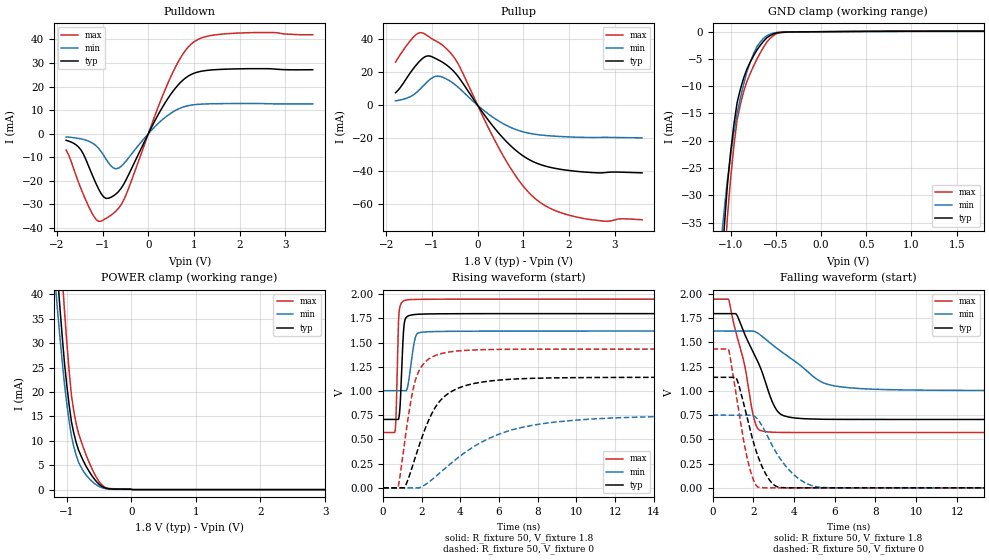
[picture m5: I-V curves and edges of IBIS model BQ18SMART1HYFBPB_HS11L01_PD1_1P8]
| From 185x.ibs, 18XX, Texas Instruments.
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|   Model Cell BQ18SMART1HYFBPB_HS11L01_PD1_1P8
|BQ18SMART1HYFBPB_HS11L01_PD1_1P8
[Model]   BQ18SMART1HYFBPB_HS11L01_PD1_1P8
Model_type   I/O
Polarity   Non-Inverting
Enable   Active-Low
Vinl =  0.63
Vinh =  1.17
Cref =  15pF
Rref =  100.0000M
Vref =  0V
Vmeas =  0.9
C_comp   0.915143p   0.8088923p   1.028577p
[Model Spec]
Vinl   0.63   0.567   0.6825
Vinh   1.17   1.053   1.2675
[Temperature Range]   25   125   -40
[Voltage Range]   1.8   1.62   1.95
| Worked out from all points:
|   slope of the pulldown table from 0 to 0.27 V, typ, clamps not added: 27.2 ohm
|   slope of the pullup table from 0 to 0.27 V, typ, clamps not added: 26 ohm
|   GND clamp passes 1 mA (typ) near -0.59 V on its own axis
|   POWER clamp passes 1 mA (typ) near -0.49 V on its own axis
|   rising waveform, R_fixture 50, V_fixture 1.8: 20-80 % time 144ps typ, 263ps min, 101ps max; typ from 0.706 V to 1.8 V
|   rising waveform, R_fixture 50, V_fixture 0: 20-80 % time 1.49ns typ, 3.72ns min, 739ps max; typ from 0 V to 1.14 V
|   falling waveform, R_fixture 50, V_fixture 1.8: 20-80 % time 1.27ns typ, 2.26ns min, 837ps max; typ from 1.8 V to 0.706 V
|   falling waveform, R_fixture 50, V_fixture 0: 20-80 % time 937ps typ, 1.39ns min, 707ps max; typ from 1.14 V to 0 V
| Nom Voltages:
|   BIASFET=1.8, VBBNW=1.1, VDD=1.1, VDDS=1.8, VSS=0, VSSS=0
| Min Voltages:
|   BIASFET=1.62, VBBNW=0.99, VDD=0.99, VDDS=1.62, VSS=0, VSSS=0
| Max Voltages:
|   BIASFET=1.95, VBBNW=1.21, VDD=1.21, VDDS=1.95, VSS=0, VSSS=0
[POWER_clamp]
|   voltage   I(typ)   I(min)   I(max)
-1.8V     196.9mA    157.5mA    250.4mA
-1.182V   51.67mA    43mA       68.61mA
-1.145V   44.45mA    37.16mA    60.1mA
-1.109V   37.9mA     31.74mA    52.07mA
-1.073V   31.79mA    26.6mA     44.33mA
-1.036V   26.12mA    21.74mA    36.87mA
-963.6mV  17.39mA    14.07mA    24.42mA
-927.3mV  13.91mA    10.96mA    19.29mA
-854.5mV  9.657mA    7.054mA    13.5mA
-709.1mV  4.995mA    3.131mA    7.393mA
-490.9mV  991uA      585.4uA    1.466mA
3.6V      0A         0A         0A
[Pulldown]
|   voltage   I(typ)   I(min)   I(max)
-1.8V     -2.835mA   -1.376mA   -6.938mA
-1.473V   -6.994mA   -2.229mA   -23.44mA
-1.2V     -18.79mA   -4.282mA   -34.89mA
-1.036V   -25.34mA   -7.531mA   -37.14mA
-872.7mV  -27.39mA   -12.36mA   -35.28mA
-654.5mV  -24.59mA   -14.63mA   -31.68mA
-490.9mV  -19.69mA   -11.65mA   -26.08mA
381.8mV   13.54mA    7.116mA    19.32mA
654.5mV   20.72mA    10.44mA    30.47mA
927.3mV   25mA       12.07mA    37.79mA
1.636V    27.3mA     12.74mA    42.26mA
3.6V      27.12mA    12.64mA    41.97mA
[Pullup]
|   voltage   I(typ)   I(min)   I(max)
-1.8V     7.614mA    2.74mA     26.22mA
-1.527V   17.69mA    4.626mA    37.43mA
-1.309V   25.69mA    8.541mA    43.72mA
-1.036V   29.87mA    15.94mA    41.05mA
-818.2mV  26.95mA    17.52mA    37.49mA
-490.9mV  19.61mA    12.45mA    28.08mA
545.5mV   -19.54mA   -10.94mA   -30.03mA
927.3mV   -29.38mA   -15.56mA   -46.58mA
1.255V    -34.7mA    -17.56mA   -56.51mA
1.691V    -38.25mA   -18.74mA   -63.85mA
2.291V    -40.42mA   -19.45mA   -68.55mA
3.6V      -41.01mA   -19.75mA   -69.5mA
[GND_clamp]
|   voltage   I(typ)   I(min)   I(max)
-1.8V     -274mA     -200.4mA   -365.5mA
-1.109V   -45.41mA   -39.33mA   -55.91mA
-1.073V   -36.49mA   -33.11mA   -44.46mA
-1.036V   -28.34mA   -27.37mA   -34.29mA
-1V       -22.19mA   -22.71mA   -27mA
-927.3mV  -12.97mA   -14.93mA   -16.12mA
-854.5mV  -8.452mA   -9.555mA   -10.93mA
-781.8mV  -5.549mA   -5.539mA   -7.634mA
-709.1mV  -3.363mA   -2.741mA   -5.028mA
-600mV    -1.121mA   -737.1uA   -1.924mA
-381.8mV  -62.21uA   -38.42uA   -93.33uA
1.8V      98.66uA    51.35uA    168.2uA
[Ramp]
| variable   typ   min   max
dV/dt_f 0.65743107/1.2769813n 0.37040169/2.2761326n  0.8285477/0.84082598n
dV/dt_r 0.69368339/1.4919074n 0.45713508/3.8126662n 0.86809185/0.74150225n
R_load = 50
[Rising Waveform]
R_fixture = 50
V_fixture = 1.8
V_fixture_min = 1.62
V_fixture_max = 1.95
|   time   V(typ)   V(min)   V(max)
0s        706.3mV    1.003V     571.6mV
615.9ps   706.3mV    1.003V     587.5mV
674.7ps   706.3mV    1.003V     786.4mV
765.6ps   706.3mV    1.003V     1.553V
813.4ps   722mV      1.003V     1.785V
1.108ns   1.715V     1.003V     1.934V
1.276ns   1.772V     1.052V     1.941V
1.65ns    1.79V      1.541V     1.945V
1.933ns   1.793V     1.605V     1.946V
17.87ns   1.798V     1.619V     1.948V
[Rising Waveform]
R_fixture = 50
V_fixture = 0
V_fixture_min = 0
V_fixture_max = 0
|   time   V(typ)   V(min)   V(max)
0s        0V         0V         0V
767.3ps   0V         0V         0V
1.102ns   0V         0V         456.7mV
1.413ns   158.8mV    0V         871.2mV
1.649ns   306.5mV    0V         1.097V
2.025ns   530.6mV    14.88mV    1.263V
2.686ns   827.2mV    111.7mV    1.365V
4.176ns   1.05V      356.5mV    1.418V
7.342ns   1.128V     630.7mV    1.431V
18.03ns   1.141V     743.9mV    1.432V
[Falling Waveform]
R_fixture = 50
V_fixture = 1.8
V_fixture_min = 1.62
V_fixture_max = 1.95
|   time   V(typ)   V(min)   V(max)
0s        1.797V     1.618V     1.947V
793.1ps   1.797V     1.618V     1.943V
1.194ns   1.784V     1.618V     1.57V
1.579ns   1.586V     1.618V     1.264V
2.025ns   1.389V     1.616V     725mV
2.342ns   1.245V     1.578V     593.1mV
3.114ns   814mV      1.447V     572.9mV
3.852ns   726.5mV    1.336V     571.2mV
6.444ns   706.2mV    1.039V     571mV
17.87ns   705.8mV    1.004V     571mV
[Falling Waveform]
R_fixture = 50
V_fixture = 0
V_fixture_min = 0
V_fixture_max = 0
|   time   V(typ)   V(min)   V(max)
0s        1.141V     750.3mV    1.432V
798.4ps   1.141V     750.3mV    1.422V
1.194ns   1.12V      750.3mV    920.4mV
1.652ns   763.7mV    750.3mV    356.9mV
1.97ns    500.8mV    748.5mV    103.7mV
2.241ns   320.2mV    700.9mV    7.064mV
3.12ns    16.65mV    366.9mV    0V
3.994ns   0V         136.2mV    0V
5.031ns   0V         14.47mV    0V
18.03ns   0V         0V         0V
